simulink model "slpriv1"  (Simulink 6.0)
settings: Solver=ode45  StartTime=0.0  StopTime=4.0  RelTol=1e-3
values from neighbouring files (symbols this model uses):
  a = 0.001    [red1m.m]    (also in slpriv1m.m; SAUAnalizeProject.m = axes( 'Parent',  centerPanel,   'Projection', 'perspective',; TESTm.m)
  ak0 = 1    [slpriv1m.m]    (also in TESTm.m)
  ak1 = 0.5    [slpriv1m.m]    (also in TESTm.m)
  ap0 = 1    [slpriv1m.m]    (also in TESTm.m)
  ap1 = 0.001    [slpriv1m.m]    (also in TESTm.m)
  bk0 = 0    [slpriv1m.m]    (also in TESTm.m)
  bk1 = 0.5    [slpriv1m.m]    (also in TESTm.m)
  bp0 = 1    [slpriv1m.m]    (also in TESTm.m)
  bp1 = 0.001    [slpriv1m.m]    (also in TESTm.m)
  c = 2000000    [red1m.m]    (also in slpriv1m.m; TESTm.m)
  F1 = 0    [red1m.m]    (also in slpriv1m.m; main5.m = peaks(35); main7.m = zeros(A1n,A2n); TESTm.m)
  F2 = 0    [red1m.m]    (also in slpriv1m.m; main5.m = membrane; main7.m = zeros(A1n,A2n); TESTm.m)
  G = 0    [red1m.m]    (also in slpriv1m.m; TESTm.m)
  G1 = 0    [red1m.m]    (also in slpriv1m.m; TESTm.m)
  G2 = 0    [red1m.m]    (also in slpriv1m.m; TESTm.m)
  i = 100    [red1m.m]    (also in slpriv1m.m; SAUAnalizeProject.m = find( isoLevel == src ); TESTm.m)
  J = 0.16    [slpriv1m.m]    (also in TESTm.m = 0.04)
  Jn = 200    [red1m.m]    (also in slpriv1m.m; TESTm.m)
  k1 = 1/R    (= 0.625)    [myparam.m]    (also in slpriv1m.m; TESTm.m = 2)
  Kc = 0.0015    [slpriv1m.m]    (also in TESTm.m)
  Ki = 0.0003    [slpriv1m.m]    (also in TESTm.m)
  kip = 0    [slpriv1m.m]    (also in TESTm.m)
  Kk = 22500    [slpriv1m.m]    (also in TESTm.m)
  km = 0.064    [myparam.m]    (also in slpriv1m.m; TESTm.m = 0.36)
  kpd = 0    [slpriv1m.m]    (also in TESTm.m)
  kpid = 1    [slpriv1m.m]    (also in TESTm.m)
  kv = 0.576    [myparam.m]    (also in slpriv1m.m; TESTm.m = 0.45)
  T = L/R    (= 0.5)    [myparam.m]    (also in slpriv1m.m; TESTm.m = 0.02)
libraries: slctrlobsolete x2

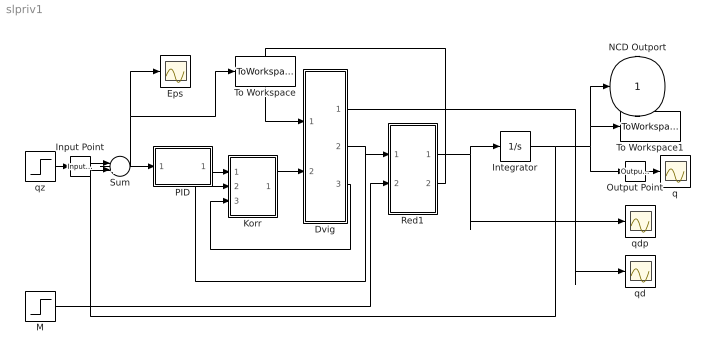
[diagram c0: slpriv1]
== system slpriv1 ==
  Dvig : Subsystem  AncestorBlock=simulink3/Signals & Systems/SubSystem
  Eps : Scope
  Input Point : slctrlobsolete/Input Point
  Integrator : Integrator
  Korr : Subsystem
  M : Step  Time=0  After=0  SampleTime=0
  Output Point : slctrlobsolete/Output Point
  PID : Subsystem
  Red1 : Subsystem
  Sum : Sum  Inputs=|+-
  To Workspace : ToWorkspace  VariableName=simouteps  SampleTime=-1  SaveFormat=Structure
  To Workspace1 : ToWorkspace  VariableName=simoutq  SampleTime=-1  SaveFormat=Structure
  q : Scope
  qd : Scope
  qdp : Scope
  qz : Step  Time=0  After=0.1  SampleTime=0
  NCD Outport : Outport  InitialOutput=0
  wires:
  Sum/1 -> PID/1(eps), Eps/1, To Workspace/1
  PID/1(ueps) -> Korr/1(u_eps)
  Red1/2(M2M) -> Dvig/1(Mv)
  Korr/1(u_d) -> Dvig/2(u)
  Dvig/2(qd') -> Red1/1(q1p), Korr/2(qdp)
  Dvig/3(ia) -> Korr/3(ia)
  M/1 -> Red1/2(-M2)
  Red1/1(q2p) -> Integrator/1, qdp/1
  Integrator/1 -> Sum/2, Output Point/1, To Workspace1/1, NCD Outport/1
  Dvig/1(qd) -> qd/1
  qz/1 -> Input Point/1
  Input Point/1 -> Sum/1
  Output Point/1 -> q/1

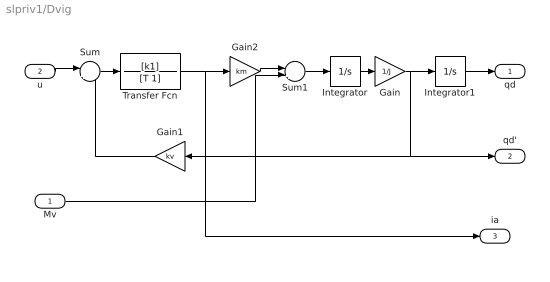
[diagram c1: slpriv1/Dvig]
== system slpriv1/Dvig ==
  Mv : Inport  Port=1  LatchInput=off
  u : Inport  Port=2  LatchInput=off
  Gain : Gain  Gain=1/J
  Gain1 : Gain  Orientation=left  Gain=kv
  Gain2 : Gain  Gain=km
  Integrator : Integrator
  Integrator1 : Integrator
  Sum : Sum  Inputs=|+-
  Sum1 : Sum  Inputs=|++
  Transfer Fcn : TransferFcn  Numerator=[k1]  Denominator=[T 1]
  qd : Outport
  qd' : Outport  Port=2
  ia : Outport  Port=3
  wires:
  u/1 -> Sum/1
  Gain1/1 -> Sum/2
  Sum/1 -> Transfer Fcn/1
  Transfer Fcn/1 -> Gain2/1, ia/1
  Gain2/1 -> Sum1/1
  Mv/1 -> Sum1/2
  Sum1/1 -> Integrator/1
  Integrator/1 -> Gain/1
  Gain/1 -> Integrator1/1, Gain1/1, qd'/1
  Integrator1/1 -> qd/1

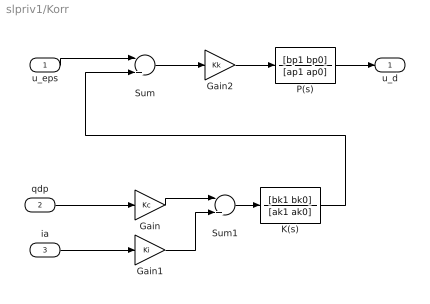
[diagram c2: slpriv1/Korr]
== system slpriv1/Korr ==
  u_eps : Inport  Port=1  LatchInput=off
  qdp : Inport  Port=2  LatchInput=off
  ia : Inport  Port=3  LatchInput=off
  Gain : Gain  Gain=Kc
  Gain1 : Gain  Gain=Ki
  Gain2 : Gain  Gain=Kk
  K(s) : TransferFcn  Numerator=[bk1 bk0]  Denominator=[ak1 ak0]
  P(s) : TransferFcn  Numerator=[bp1 bp0]  Denominator=[ap1 ap0]
  Sum : Sum  Inputs=|+-
  Sum1 : Sum  Inputs=|++
  u_d : Outport
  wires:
  u_eps/1 -> Sum/1
  qdp/1 -> Gain/1
  ia/1 -> Gain1/1
  Sum/1 -> Gain2/1
  Gain/1 -> Sum1/1
  Gain1/1 -> Sum1/2
  Gain2/1 -> P(s)/1
  P(s)/1 -> u_d/1
  Sum1/1 -> K(s)/1
  K(s)/1 -> Sum/2

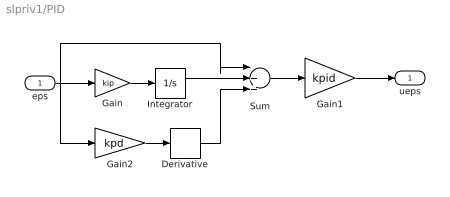
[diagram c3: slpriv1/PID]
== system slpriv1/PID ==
  eps : Inport  Port=1  LatchInput=off
  Derivative : Derivative
  Gain : Gain  Gain=kip
  Gain1 : Gain  Gain=kpid
  Gain2 : Gain  Gain=kpd
  Integrator : Integrator
  Sum : Sum  Inputs=|+++
  ueps : Outport
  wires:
  Gain1/1 -> ueps/1
  Sum/1 -> Gain1/1
  Gain/1 -> Integrator/1
  eps/1 -> Gain/1, Sum/1, Gain2/1
  Integrator/1 -> Sum/2
  Gain2/1 -> Derivative/1
  Derivative/1 -> Sum/3

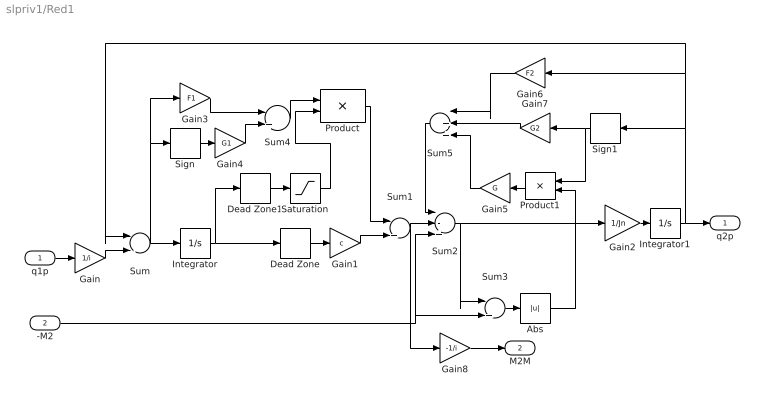
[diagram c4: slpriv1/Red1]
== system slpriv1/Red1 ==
  q1p : Inport  Port=1  LatchInput=off
  -M2 : Inport  Port=2  LatchInput=off
  Abs : Abs
  Dead Zone : DeadZone  LowerValue=-a  UpperValue=a
  Dead Zone1 : DeadZone  LowerValue=-a  UpperValue=a
  Gain : Gain  Gain=1/i
  Gain1 : Gain  Gain=c
  Gain2 : Gain  Gain=1/Jn
  Gain3 : Gain  Gain=F1
  Gain4 : Gain  Gain=G1
  Gain5 : Gain  Orientation=left  Gain=G
  Gain6 : Gain  Orientation=left  Gain=F2
  Gain7 : Gain  Orientation=left  Gain=G2
  Gain8 : Gain  Gain=-1/i
  Integrator : Integrator
  Integrator1 : Integrator
  Product : Product
  Product1 : Product  Orientation=left
  Saturation : Saturate  UpperLimit=a  LowerLimit=-a
  Sign : Signum
  Sign1 : Signum  Orientation=left
  Sum : Sum  Inputs=|-+
  Sum1 : Sum  Inputs=|++
  Sum2 : Sum  Inputs=|-++
  Sum3 : Sum  Inputs=|++
  Sum4 : Sum  Inputs=|++
  Sum5 : Sum  Orientation=left  Inputs=|+++
  q2p : Outport
  M2M : Outport  Port=2
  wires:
  q1p/1 -> Gain/1
  Gain/1 -> Sum/2
  Sum/1 -> Integrator/1, Gain3/1, Sign/1
  Integrator/1 -> Dead Zone/1, Dead Zone1/1
  Dead Zone/1 -> Gain1/1
  Gain1/1 -> Sum1/2
  Sum1/1 -> Sum2/2, Gain8/1
  Sum2/1 -> Gain2/1, Sum3/1
  Gain2/1 -> Integrator1/1
  Integrator1/1 -> q2p/1, Sign1/1, Gain6/1, Sum/1
  -M2/1 -> Sum3/2, Sum2/3
  Sum3/1 -> Abs/1
  Gain3/1 -> Sum4/1
  Gain4/1 -> Sum4/2
  Sign/1 -> Gain4/1
  Sum4/1 -> Product/1
  Product/1 -> Sum1/1
  Sum5/1 -> Sum2/1
  Product1/1 -> Gain5/1
  Gain5/1 -> Sum5/3
  Abs/1 -> Product1/2
  Gain6/1 -> Sum5/1
  Gain7/1 -> Sum5/2
  Sign1/1 -> Gain7/1, Product1/1
  Gain8/1 -> M2M/1
  Dead Zone1/1 -> Saturation/1
  Saturation/1 -> Product/2
